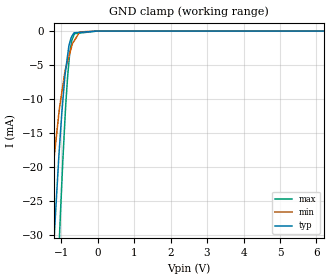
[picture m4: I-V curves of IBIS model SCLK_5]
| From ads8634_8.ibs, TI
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|   SCLK_5   5V digital input Model
[Model] SCLK_5   | 5V digital input
Model_type Input
Vinl = 1.5
Vinh = 3.5
|   typ   min   max
|   (nom PVT)   (Fast PVT)   (slow PVT)
|C_comp from L-C Tank method(L=1nH)
|Resonant Frequency(Hz)  3.97G   4.29G   3.78G
C_comp   1.60724E-12   1.3807E-12   1.77861E-12
| Where   nom PVT is  Nominal Process, 5V, 25C
|   Fast PVT is Strong Process, 4.5V, -40C
|   Slow PVT is Weak Process, 5.5V, 85C
|C_comp - from L-C Tank method, L = 1nH, peak frequency
[Model Spec]   | 5V
Vinl   1.5   1.35   1.65
Vinh   3.5   3.15   3.85
|Vinl = 0.3 DVDD
|Vinh = 0.7 DVDD
[Voltage Range]   5   4.75   5.25
[Temperature Range]   27   125   -40
[Power Clamp Reference]   5   4.75   5.25
[GND Clamp Reference]   0   0   0
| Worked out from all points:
|   GND clamp passes 1 mA (typ) near -0.73 V on its own axis
[GND Clamp]
|   Voltage   I(typ)   I(min)   I(max)
-5V       -508.3mA   -353.4mA   -632.6mA
-1.379V   -49.44mA   -29.14mA   -77.53mA
-1.244V   -35.28mA   -21.21mA   -57.61mA
-1.127V   -24.36mA   -15.32mA   -40.99mA
-1.05V    -17.41mA   -11.49mA   -30.85mA
-1.034V   -16.14mA   -10.91mA   -28.69mA
-907.5mV  -7.26mA    -6.389mA   -14.3mA
-821.9mV  -3.577mA   -4.411mA   -6.679mA
-757.8mV  -1.589mA   -3.167mA   -2.995mA
-644.5mV  -249.2uA   -1.463mA   -511.6uA
-23.21mV  0A         0A         -4.793uA
9.985V    0A         0A         0A
[POWER Clamp]
|   SCR cell for ESD function. Effects occurr above VDD x 2
|   Voltage   I(typ)   I(min)   I(max)
-5V       0A         0A         0A
0V        0A         0A         0A
10V       0A         0A         0A
